| TEXAS INSTRUMENTS INCORPORATED
| Standard Linear and Logic Group
| IBIS Model of MAX3243E
| 3-V TO 5.5-V MULTICHANNEL RS-232 LINE DRIVER/RECEIVER WITH +-15 kV
| IEC ESD PROTECTION
| This file contains package information for the following:
|  TSSOP 28-pin (PW) package as [Component] MAXE3243L_PW
|  SSOP 28-pin (DB) package as [Component] MAXE3243L_DB
|  SOIC 28-pin (DW) package as [Component] MAXE3243L_DW
|  QFN 32-PIN (RHB) package as [Component] MAX3243E_RHB
| This device can be powered at the following Vccs:
|  5 volt Vcc
|  3.3 volt Vcc
| This file provides unique models under the [Model Selector] for each Vcc.
| For operation at a specific Vcc, select the appropriate model after each
| [Model Selector] keyword.
[IBIS Ver]   3.2
[Comment char]  |_char
[File Name]   max3243e.ibs
[File Rev]   1.1 | l_die
[Date]   August 23, 2007
[Source]   Data created from TI-SPICE simulations at TI-SLL.
[Notes]   The following is an IBIS list for the MAX3243E.
   Please contact sllibis@ti.com with questions and
   comments concerning SLL IBIS models.
   - We violated the sweep range for receiver input and
   driver output assuming that there will be no reflection
   issue in practice.
   - Since the receiver of RS-232 has no Vinl and Vinh, we
   omitted those parameters
   - Since receiver input has input resistor conected to ground
   the receiver input power clamp data does not go to zero.
   - End point warning due to AC and DC mismatch.
   - FILE REV HISTORY
   - 1.0 RELEASE IBIS FILE ON 08/29/2007
   - 1.1 RHB package added on 09/06/2007
[Disclaimer] Property of Texas Instruments Incorporated.  Unauthorized
   reproduction and/or distribution is strictly prohibited.
   This product is protected under copyright law.
   Created  2007, (C) Copyright  2007, Texas Instruments
   Incorporated, All Rights Reserved
   UNLESS THERE IS A SIGNED, WRITTEN AGREEMENT TO THE
   CONTRARY, TEXAS INSTRUMENTS (TI) IS PROVIDING THE IBIS
   MODELS  AND WITHOUT ANY WARRANTY, EXPRESSED OR
   IMPLIED.  TI assumes no liability for:
   1) the accuracy of the IBIS models provided to your
   company;
   2) the proper functioning of these IBIS Models in your
   design or for any resulting applications; or
   3) infringement of patents, copyrights or intellectual
   property rights resulting from your use of these IBIS
   models.
   TI provides IBIS Models as a service to our customers.
   You and your company shall not distribute, sell or give
   these models to anyone else without prior written
   permission from TI.
   TI reserves the right to make changes to our products or
   to discontinue any semiconductor product or service
   without notice, and advises our customers to obtain the
   latest version of relevant information to verify, before
   placing orders, that the information being relied on is
   current.
   Please be aware that your receipt and use of the IBIS
   information provided shall serve as acceptance of these
   terms and conditions.  If you do not accept these terms,
   you should return or destroy the IBIS models and any
   other accompanying information immediately.
| Component MAX3243E_DB 28-PIN SSOP
[Component]   MAX3243E_DB
[Manufacturer]   Texas Instruments, Inc.
[Package]
|   typ   min   max
R_pkg   4.200e-02   4.000e-02   4.600e-02
L_pkg   3.658e-09   2.974e-09   4.781e-09
C_pkg   3.910e-13   2.690e-13   5.360e-13
[Pin]   signal_name   model_name   R_pin   L_pin   C_pin
1   C2+   POWER   4.600e-02   4.781e-09   5.290e-13
2   C2-   POWER   4.300e-02   4.230e-09   5.110e-13
3   VMINUS   POWER   4.200e-02   4.224e-09   5.360e-13
4   RIN1   MAX3243E_RIN   4.000e-02   3.305e-09   3.320e-13
5   RIN2   MAX3243E_RIN   4.000e-02   3.087e-09   2.890e-13
6   RIN3   MAX3243E_RIN   4.000e-02   3.004e-09   2.780e-13
7   RIN4   MAX3243E_RIN   4.100e-02   2.974e-09   2.690e-13
8   RIN5   MAX3243E_RIN   4.100e-02   2.974e-09   2.690e-13
9   DOUT1   MAX3243E_DOUT   4.000e-02   3.004e-09   2.780e-13
10   DOUT2   MAX3243E_DOUT   4.000e-02   3.086e-09   2.890e-13
11   DOUT3   MAX3243E_DOUT   4.000e-02   3.304e-09   3.320e-13
12   DIN3   MAX3243E_DIN   4.200e-02   4.224e-09   5.360e-13
13   DIN2   MAX3243E_DIN   4.300e-02   4.230e-09   5.110e-13
14   DIN1   MAX3243E_DIN   4.600e-02   4.781e-09   5.180e-13
15   ROUT5   MAX3243E_ROUT   4.600e-02   4.781e-09   5.180e-13
16   ROUT4   MAX3243E_ROUT   4.300e-02   4.229e-09   5.110e-13
17   ROUT3   MAX3243E_ROUT   4.200e-02   4.223e-09   5.360e-13
18   ROUT2   MAX3243E_ROUT   4.000e-02   3.305e-09   3.320e-13
19   ROUT1   MAX3243E_ROUT   4.000e-02   3.087e-09   2.890e-13
20   ROUT2B   MAX3243E_RBOUT   4.000e-02   3.004e-09   2.780e-13
21   INVALID   MAX3243E_RBOUT   4.100e-02   2.974e-09   2.690e-13
22   FORCEOFF   MAX3243E_FIN   4.100e-02   2.974e-09   2.690e-13
23   FORCEON   MAX3243E_FIN   4.000e-02   3.003e-09   2.780e-13
24   C1-   POWER   4.000e-02   3.086e-09   2.890e-13
25   GND   GND   4.000e-02   3.305e-09   3.310e-13
26   VCC   POWER   4.200e-02   4.224e-09   5.360e-13
27   VPLUS   POWER   4.300e-02   4.230e-09   5.110e-13
28   C1+   POWER   4.600e-02   4.781e-09   5.290e-13
| Component MAX3243E_DW 28-PIN SOIC
[Component]   MAX3243E_DW
[Manufacturer]   Texas Instruments, Inc.
[Package]
|   typ   min   max
R_pkg   3.700e-02   3.100e-02   4.600e-02
L_pkg   5.147e-09   3.554e-09   7.390e-09
C_pkg   8.040e-13   3.820e-13   1.314e-12
[Pin]   signal_name   model_name   R_pin   L_pin   C_pin
1   C2+   POWER   4.500e-02   7.390e-09   1.122e-12
2   C2-   POWER   4.300e-02   6.387e-09   1.048e-12
3   VMINUS   POWER   3.800e-02   5.461e-09   8.240e-13
4   RIN1   MAX3243E_RIN   3.700e-02   4.759e-09   5.730e-13
5   RIN2   MAX3243E_RIN   3.100e-02   4.604e-09   5.090e-13
6   RIN3   MAX3243E_RIN   3.200e-02   3.891e-09   4.580e-13
7   RIN4   MAX3243E_RIN   3.400e-02   3.554e-09   3.820e-13
8   RIN5   MAX3243E_RIN   3.400e-02   3.555e-09   3.820e-13
9   DOUT1   MAX3243E_DOUT   3.200e-02   3.891e-09   4.580e-13
10   DOUT2   MAX3243E_DOUT   3.100e-02   4.604e-09   5.090e-13
11   DOUT3   MAX3243E_DOUT   3.300e-02   4.744e-09   5.730e-13
12   DIN3   MAX3243E_DIN   3.600e-02   5.454e-09   8.240e-13
13   DIN2   MAX3243E_DIN   4.200e-02   6.382e-09   1.049e-12
14   DIN1   MAX3243E_DIN   4.600e-02   7.383e-09   1.074e-12
15   ROUT5   MAX3243E_ROUT   4.600e-02   7.383e-09   1.266e-12
16   ROUT4   MAX3243E_ROUT   4.200e-02   6.382e-09   1.262e-12
17   ROUT3   MAX3243E_ROUT   3.600e-02   5.454e-09   1.037e-12
18   ROUT2   MAX3243E_ROUT   3.300e-02   4.744e-09   7.870e-13
19   ROUT1   MAX3243E_ROUT   3.100e-02   4.604e-09   7.230e-13
20   ROUT2B   MAX3243E_RBOUT   3.200e-02   3.891e-09   6.710e-13
21   INVALID   MAX3243E_RBOUT   3.400e-02   3.554e-09   5.960e-13
22   FORCEOFF   MAX3243E_FIN   3.400e-02   3.554e-09   5.960e-13
23   FORCEON   MAX3243E_FIN   3.200e-02   3.891e-09   6.710e-13
24   C1-   POWER   3.100e-02   4.604e-09   7.230e-13
25   GND   GND   3.700e-02   4.759e-09   7.870e-13
26   VCC   POWER   3.800e-02   5.461e-09   1.037e-12
27   VPLUS   POWER   4.300e-02   6.387e-09   1.261e-12
28   C1+   POWER   4.500e-02   7.390e-09   1.314e-12
| Component MAX3243E_PW 28-PIN TSSOP
[Component]   MAX3243E_PW
[Manufacturer]   Texas Instruments, Inc.
[Package]
|   typ   min   max
R_pkg   2.300e-02   1.900e-02   3.000e-02
L_pkg   1.781e-09   1.295e-09   2.916e-09
C_pkg   1.390e-13   7.700e-14   3.160e-13
[Pin]   signal_name   model_name   R_pin   L_pin   C_pin
1   C2+   POWER   3.000e-02   2.916e-09   3.160e-13
2   C2-   POWER   2.900e-02   2.409e-09   1.910e-13
3   VMINUS   POWER   2.500e-02   1.805e-09   1.400e-13
4   RIN1   MAX3243E_RIN   2.000e-02   1.336e-09   9.200e-14
5   RIN2   MAX3243E_RIN   2.000e-02   1.329e-09   8.000e-14
6   RIN3   MAX3243E_RIN   2.100e-02   1.360e-09   7.900e-14
7   RIN4   MAX3243E_RIN   2.100e-02   1.359e-09   7.900e-14
8   RIN5   MAX3243E_RIN   2.100e-02   1.343e-09   7.800e-14
9   DOUT1   MAX3243E_DOUT   2.000e-02   1.327e-09   7.800e-14
10   DOUT2   MAX3243E_DOUT   2.100e-02   1.345e-09   8.000e-14
11   DOUT3   MAX3243E_DOUT   2.000e-02   1.335e-09   9.200e-14
12   DIN3   MAX3243E_DIN   2.500e-02   1.799e-09   1.420e-13
13   DIN2   MAX3243E_DIN   2.600e-02   2.338e-09   1.890e-13
14   DIN1   MAX3243E_DIN   2.800e-02   2.878e-09   3.140e-13
15   ROUT5   MAX3243E_ROUT   3.000e-02   2.910e-09   3.140e-13
16   ROUT4   MAX3243E_ROUT   2.900e-02   2.431e-09   1.910e-13
17   ROUT3   MAX3243E_ROUT   2.700e-02   1.903e-09   1.450e-13
18   ROUT2   MAX3243E_ROUT   1.900e-02   1.319e-09   9.100e-14
19   ROUT1   MAX3243E_ROUT   1.900e-02   1.313e-09   7.900e-14
20   ROUT2B   MAX3243E_RBOUT   2.000e-02   1.327e-09   7.800e-14
21   INVALID   MAX3243E_RBOUT   2.000e-02   1.327e-09   7.800e-14
22   FORCEOFF   MAX3243E_FIN   1.900e-02   1.295e-09   7.700e-14
23   FORCEON   MAX3243E_FIN   2.000e-02   1.327e-09   7.800e-14
24   C1-   POWER   2.000e-02   1.328e-09   8.000e-14
25   GND   GND   2.000e-02   1.335e-09   9.200e-14
26   VCC   POWER   2.700e-02   1.894e-09   1.450e-13
27   VPLUS   POWER   2.700e-02   2.397e-09   1.900e-13
28   C1+   POWER   2.900e-02   2.892e-09   3.140e-13
| Component MAX3243E_RHB 32-PIN QFN
[Component]   MAX3243E_RHB
[Manufacturer]   Texas Instruments, Inc.
[Package]
|   typ   min   max
R_pkg   8.871e-02   1.120e-03   1.231e-01
L_pkg   1.225e-09   1.303e-10   1.699e-09
C_pkg   1.629e-13   8.116e-14   1.935e-13
[Pin]   signal_name   model_name   R_pin   L_pin   C_pin
1   RIN1   MAX3243E_RIN   1.176e-01   1.631e-09   1.732e-13
2   RIN2   MAX3243E_RIN   1.142e-01   1.575e-09   1.874e-13
3   RIN3   MAX3243E_RIN   1.130e-01   1.556e-09   1.863e-13
4   RIN4   MAX3243E_RIN   1.129e-01   1.554e-09   1.862e-13
5   RIN5   MAX3243E_RIN   1.139e-01   1.569e-09   1.866e-13
6   DOUT1   MAX3243E_DOUT   1.152e-01   1.588e-09   1.877e-13
7   DOUT2   MAX3243E_DOUT   1.177e-01   1.626e-09   1.902e-13
8   DOUT3   MAX3243E_DOUT   1.221e-01   1.698e-09   1.759e-13
9   NC   NC   1.120e-03   1.303e-10   8.118e-14
10   DIN3   MAX3243E_DIN   9.388e-02   1.275e-09   1.712e-13
11   DIN2   MAX3243E_DIN   8.243e-02   1.108e-09   1.636e-13
12   DIN1   MAX3243E_DIN   7.524e-02   1.005e-09   1.557e-13
13   ROUT5   MAX3243E_ROUT   7.328e-02   9.760e-10   1.528e-13
14   ROUT4   MAX3243E_ROUT   7.563e-02   1.008e-09   1.545e-13
15   ROUT3   MAX3243E_ROUT   8.250e-02   1.105e-09   1.598e-13
16   NC   NC   1.120e-03   1.303e-10   8.116e-14
17   ROUT2   MAX3243E_ROUT   1.190e-01   1.643e-09   1.744e-13
18   ROUT1   MAX3243E_ROUT   1.142e-01   1.566e-09   1.884e-13
19   ROUT2B   MAX3243E_RBOUT   1.111e-01   1.518e-09   1.861e-13
20   INVALID   MAX3243E_RBOUT   1.105e-01   1.510e-09   1.834e-13
21   FORCEOFF   MAX3243E_FIN   1.121e-01   1.533e-09   1.857e-13
22   FORCEON   MAX3243E_FIN   1.132e-01   1.550e-09   1.888e-13
23   C1-   POWER   1.231e-01   1.699e-09   1.935e-13
24   GND   GND   1.169e-01   1.612e-09   1.729e-13
25   NC   NC   1.120e-03   1.303e-10   8.117e-14
26   VCC   POWER   8.785e-02   1.181e-09   1.667e-13
27   VPLUS   POWER   8.270e-02   1.107e-09   1.621e-13
28   C1+   POWER   7.803e-02   1.042e-09   1.584e-13
29   C2+   POWER   7.800e-02   1.043e-09   1.584e-13
30   C2-   POWER   8.323e-02   1.119e-09   1.641e-13
31   VMINUS   POWER   9.487e-02   1.289e-09   1.731e-13
32   NC   NC   1.120e-03   1.303e-10   8.116e-14
| Model MAX3243E_DIN
[Model Selector]   MAX3243E_DIN
MAX3243E_DIN_50   5 volt Vcc
MAX3243E_DIN_33   3.3 volt Vcc
| Model MAX3243E_FIN
[Model Selector]   MAX3243E_FIN
MAX3243E_FIN_50   5 volt Vcc
MAX3243E_FIN_33   3.3 volt Vcc
| Model MAX3243E_RIN
[Model Selector]   MAX3243E_RIN
MAX3243E_RIN_50   5 volt Vcc
MAX3243E_RIN_33   3.3 volt Vcc
| Model MAX3243E_RBOUT
[Model Selector]   MAX3243E_RBOUT
MAX3243E_RBOUT_50   5 volt Vcc
MAX3243E_RBOUT_33   3.3 volt Vcc
| Model MAX3243E_ROUT
[Model Selector]   MAX3243E_ROUT
MAX3243E_ROUT_50   5 volt Vcc
MAX3243E_ROUT_33   3.3 volt Vcc
| Model MAX3243E_DOUT
[Model Selector]   MAX3243E_DOUT
MAX3243E_DOUT_50   5 volt Vcc
MAX3243E_DOUT_33   3.3 volt Vcc
| Models and submodels in the file (12): MAX3243E_RIN_50 (Input), MAX3243E_RIN_33 (Input), MAX3243E_DIN_50 (Input), MAX3243E_DIN_33 (Input), MAX3243E_FIN_50 (Input), MAX3243E_FIN_33 (Input), MAX3243E_RBOUT_50 (Output), MAX3243E_RBOUT_33 (Output), MAX3243E_ROUT_50 (3-state), MAX3243E_ROUT_33 (3-state), MAX3243E_DOUT_50 (3-state), MAX3243E_DOUT_33 (3-state)
